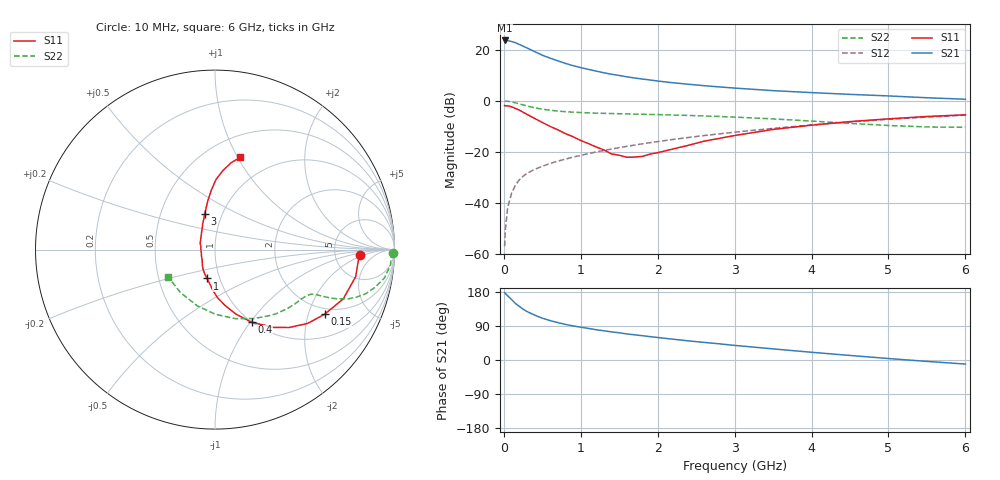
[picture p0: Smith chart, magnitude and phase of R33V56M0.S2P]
! SIEMENS Small Signal Semiconductors
! BFR181
! Si NPN RF Bipolar Junction Transistor in SOT23
! VCE = 3.5 V  IC = 6 mA
! Common Emitter S-Parameters:  May  1996
# GHz  S  MA  R  50
!  f  S11  S21  S12  S22
! GHz  MAG  ANG  MAG  ANG  MAG  ANG  MAG  ANG
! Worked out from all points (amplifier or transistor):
!   36 points, 10 MHz to 6 GHz, reference 50 ohm
!   highest |S21| = 23.7 dB at 10 MHz (marker M1)
!   |S21| within 3 dB of that: start of sweep to 304.1 MHz
!   unconditionally stable (mu >= 1): 1.013 GHz to 2.866 GHz
!   at 250 MHz: K = 0.46, MSG = 25.6 dB, |S12| = -29.6 dB
!   at 1.4 GHz: K = 1.05, MAG = 13.3 dB, |S12| = -18.9 dB
!   at 6 GHz: K = 0.85, MSG = 3.1 dB, |S12| = -5.6 dB
!   S11 on the Smith chart (normalised r, x): 10 MHz: 9.21, -1.66; 150 MHz: 1.77, -2.56; 400 MHz: 1.00, -1.01; 1 GHz: 0.87, -0.29; 3 GHz: 0.83, +0.35; 6 GHz: 0.71, +1.02
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0.01  0.8097 -2.2  15.37 177.7  0.0014 91.7  0.9911 -1.0
0.02  0.801 -4.2  15.36 175.4  0.003 89.5  0.9839 -2.0
0.05  0.7982 -10.9  15.27 169.4  0.008 84.9  0.9816 -5.0
0.1  0.7656 -21.0  14.65 159.6  0.0153 80.8  0.9574 -9.5
0.15  0.7094 -30.5  13.89 149.3  0.0219 75.3  0.9143 -13.4
0.2  0.6603 -38.5  12.88 141.6  0.028 72.1  0.8739 -16.4
0.25  0.5993 -46.4  11.88 134.2  0.0331 68.8  0.8331 -18.5
0.3  0.5436 -52.9  10.95 128.0  0.0376 67.4  0.7934 -20.2
0.4  0.4529 -63.3  9.277 118.6  0.0452 65.9  0.7321 -22.0
0.5  0.3765 -72.2  7.889 110.4  0.0518 64.7  0.6875 -22.9
0.6  0.3161 -79.8  6.919 104.0  0.059 64.7  0.6552 -23.4
0.8  0.2276 -93.0  5.449 94.0  0.0717 65.0  0.6128 -24.0
1  0.1667 -105.6  4.497 86.5  0.085 65.6  0.5903 -24.9
1.1  0.1448 -113.9  4.151 83.3  0.0921 65.8  0.5818 -25.6
1.3  0.1089 -130.4  3.565 77.1  0.1062 65.9  0.5687 -27.1
1.6  0.0779 -169.4  2.965 68.8  0.1279 65.7  0.5539 -29.8
2.2  0.1137 132.1  2.266 54.9  0.1748 63.6  0.5275 -37.0
3  0.2087 105.8  1.783 38.5  0.2426 58.4  0.4802 -49.7
3.5  0.2747 98.4  1.588 29.3  0.2883 54.4  0.4424 -60.2
4.5  0.3917 89.1  1.341 12.0  0.3858 43.8  0.3609 -89.5
5.5  0.4933 79.4  1.151 -3.7  0.4809 31.1  0.3075 -128.4
6  0.5324 74.7  1.077 -10.7  0.5247 24.2  0.3024 -149.9
